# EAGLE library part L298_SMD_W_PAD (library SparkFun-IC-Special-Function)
Full-bridge power driver IC This device uses the ground pad under the IC
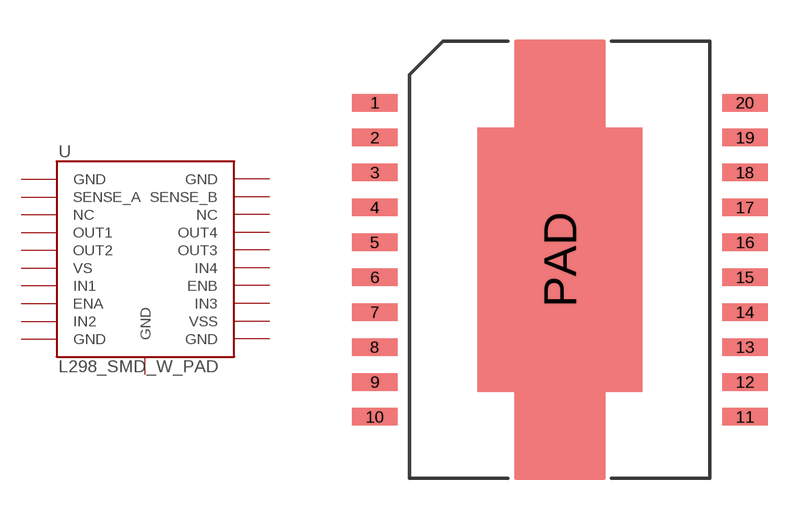
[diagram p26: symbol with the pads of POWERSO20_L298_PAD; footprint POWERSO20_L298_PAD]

Designator prefix -

## L298_SMD_W_PAD (PROD_ID: IC-09133; VALUE: L298)  [POWERSO20_L298_PAD]
1  GND
2  SENSE_A
3  NC
4  OUT1
5  OUT2
6  VS
7  IN1
8  ENA
9  IN2
10  GND
11  GND
12  VSS
13  IN3
14  ENB
15  IN4
16  OUT3
17  OUT4
18  NC
19  SENSE_B
20  GND
PAD  GND

## Footprint POWERSO20_L298_PAD (pad centres in mm)
smd 1.651 x 0.635: 1 -6.731,5.715; 2 -6.731,4.445; 3 -6.731,3.175; 4 -6.731,1.905; 5 -6.731,0.635; 6 -6.731,-0.635; 7 -6.731,-1.905; 8 -6.731,-3.175; 9 -6.731,-4.445; 10 -6.731,-5.715; 11 6.731,-5.715; 12 6.731,-4.445; 13 6.731,-3.175; 14 6.731,-1.905; 15 6.731,-0.635; 16 6.731,0.635; 17 6.731,1.905; 18 6.731,3.175; 19 6.731,4.445; 20 6.731,5.715
smd 5.994 x 9.601: PAD 0,0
